TEXTLIST question
  1 = '确定要删除当前配方文件吗?' | chinese: '确定要删除当前配方文件吗?' | english: 'Are you sure you want to delete current recipe file?'
  2 = '确认要上载并激活当前配方文件吗?' | chinese: '确认要上载并激活当前配方文件吗?' | english: 'Are you sure you want to upload and active current recipe file?'
  3 = '确认要替换当前配方文件吗(已有同名配方)?' | chinese: '确认要替换当前配方文件吗(已有同名配方)?' | english: 'Are you sure you want to replace current recipe file?'
  10 = '确认要从USB中导入配方文件吗?' | chinese: '确认要从USB中导入配方文件吗?' | english: 'Are you sure you want to import recipe file from USB device?'
  11 = '确认要复制并替换掉目标文件夹的同名文件吗?' | chinese: '确认要复制并替换掉目标文件夹的同名文件吗?' | english: 'Are you sure you want to copy and replace the file in the dest folder?'
  12 = '' | english: '12'
  20 = '确认要把文件导出到USB中吗?' | chinese: '确认要把文件导出到USB中吗?' | english: 'Are you sure you want to export recipe file to USB device?'
  21 = '确认要复制并替换掉目标文件夹的同名文件吗?' | chinese: '确认要复制并替换掉目标文件夹的同名文件吗?' | english: 'Are you sure you want to copy and replace the file in the dest folder?'
  22 = '' | english: '22'
  30 = '没有发现USB设备' | chinese: '没有发现USB设备' | english: 'No USB device.'
   = ''
END_TEXTLIST
